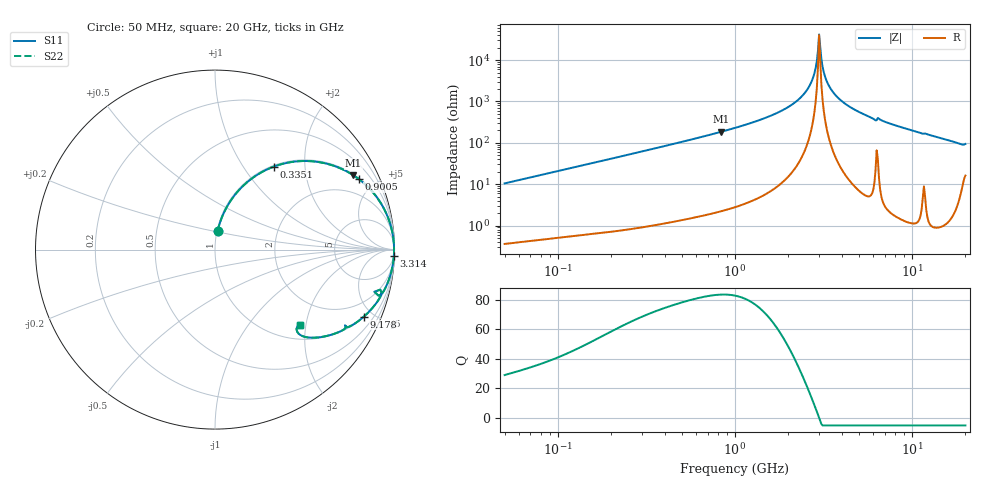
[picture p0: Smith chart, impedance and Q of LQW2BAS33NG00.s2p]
!Murata Part Number: LQW2BAS33NG00
!These Parameters are Measured in Series Mode Connection
!  o--[Z]--o
!Port1  Port2
!  o-------o
!Freq. Start=50[MHz] Stop=20[GHz], 401[Steps]
# Hz S RI R 50
!Freq.(Hz) S11(Real) S11(Imag) S21(Real) S21(Imag) S12(Real) S12(Imag) S22(Real) S22(Imag)
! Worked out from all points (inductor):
!   401 points, 50 MHz to 20 GHz, reference 50 ohm
!   read as one part in series: L = 33.1 nH near 51.52 MHz
!   highest Q = 83.5 at 835.5 MHz (marker M1), where L = 35.2 nH
!   self-resonance near 2.985 GHz
!   S11 on the Smith chart (normalised r, x): 50 MHz: 1.01, +0.21; 335.1 MHz: 1.02, +1.39; 900.5 MHz: 1.05, +4.04; 3.314 GHz: 5, -59; 9.178 GHz: 1.03, -4.44; 20 GHz: 1.32, -1.85
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5e7  0.0142 0.1025  0.9858 -0.1025  0.9858 -0.1025  0.0142 0.1025
1.364002e8  0.0782 0.2583  0.9218 -0.2583  0.9218 -0.2583  0.0782 0.2583
3.350611e8  0.3283 0.4626  0.6717 -0.4626  0.6717 -0.4626  0.3283 0.4626
3.721004e8  0.3764 0.4777  0.6236 -0.4777  0.6236 -0.4777  0.3764 0.4777
8.354841e8  0.7708 0.4144  0.2292 -0.4144  0.2292 -0.4144  0.7708 0.4144
9.00459e8  0.8001 0.394  0.1999 -0.394  0.1999 -0.394  0.8001 0.394
1e9  0.8374 0.363  0.1626 -0.363  0.1626 -0.363  0.8374 0.363
2.021818e9  0.9802 0.129  0.0198 -0.129  0.0198 -0.129  0.9802 0.129
2.419936e9  0.9926 0.0694  0.00738 -0.0694  0.00738 -0.0694  0.9926 0.0694
2.728004e9  0.9967 0.0301  0.0033 -0.0301  0.0033 -0.0301  0.9967 0.0301
2.810964e9  0.9972 0.0202  0.00278 -0.0202  0.00278 -0.0202  0.9972 0.0202
2.940159e9  0.9976 0.00551  0.00236 -0.00551  0.00236 -0.00551  0.9976 0.00551
2.98453e9  0.9977 0.000595  0.00232 -0.000595  0.00232 -0.000595  0.9977 0.000595
3.075291e9  0.9976 -0.00923  0.00238 0.00923  0.00238 0.00923  0.9976 -0.00923
3.168813e9  0.9974 -0.0191  0.00264 0.0191  0.00264 0.0191  0.9974 -0.0191
3.314454e9  0.9966 -0.0338  0.0034 0.0338  0.0034 0.0338  0.9966 -0.0338
3.680849e9  0.9931 -0.0684  0.00692 0.0684  0.00692 0.0684  0.9931 -0.0684
4.34015e9  0.9823 -0.1235  0.0177 0.1235  0.0177 0.1235  0.9823 -0.1235
7.442007e9  0.8952 -0.3027  0.1048 0.3027  0.1048 0.3027  0.8952 -0.3027
9.178299e9  0.83 -0.3728  0.17 0.3728  0.17 0.3728  0.83 -0.3728
1.573793e10  0.5814 -0.4886  0.4186 0.4886  0.4186 0.4886  0.5814 -0.4886
2e10  0.4733 -0.4196  0.5267 0.4196  0.5267 0.4196  0.4733 -0.4196
